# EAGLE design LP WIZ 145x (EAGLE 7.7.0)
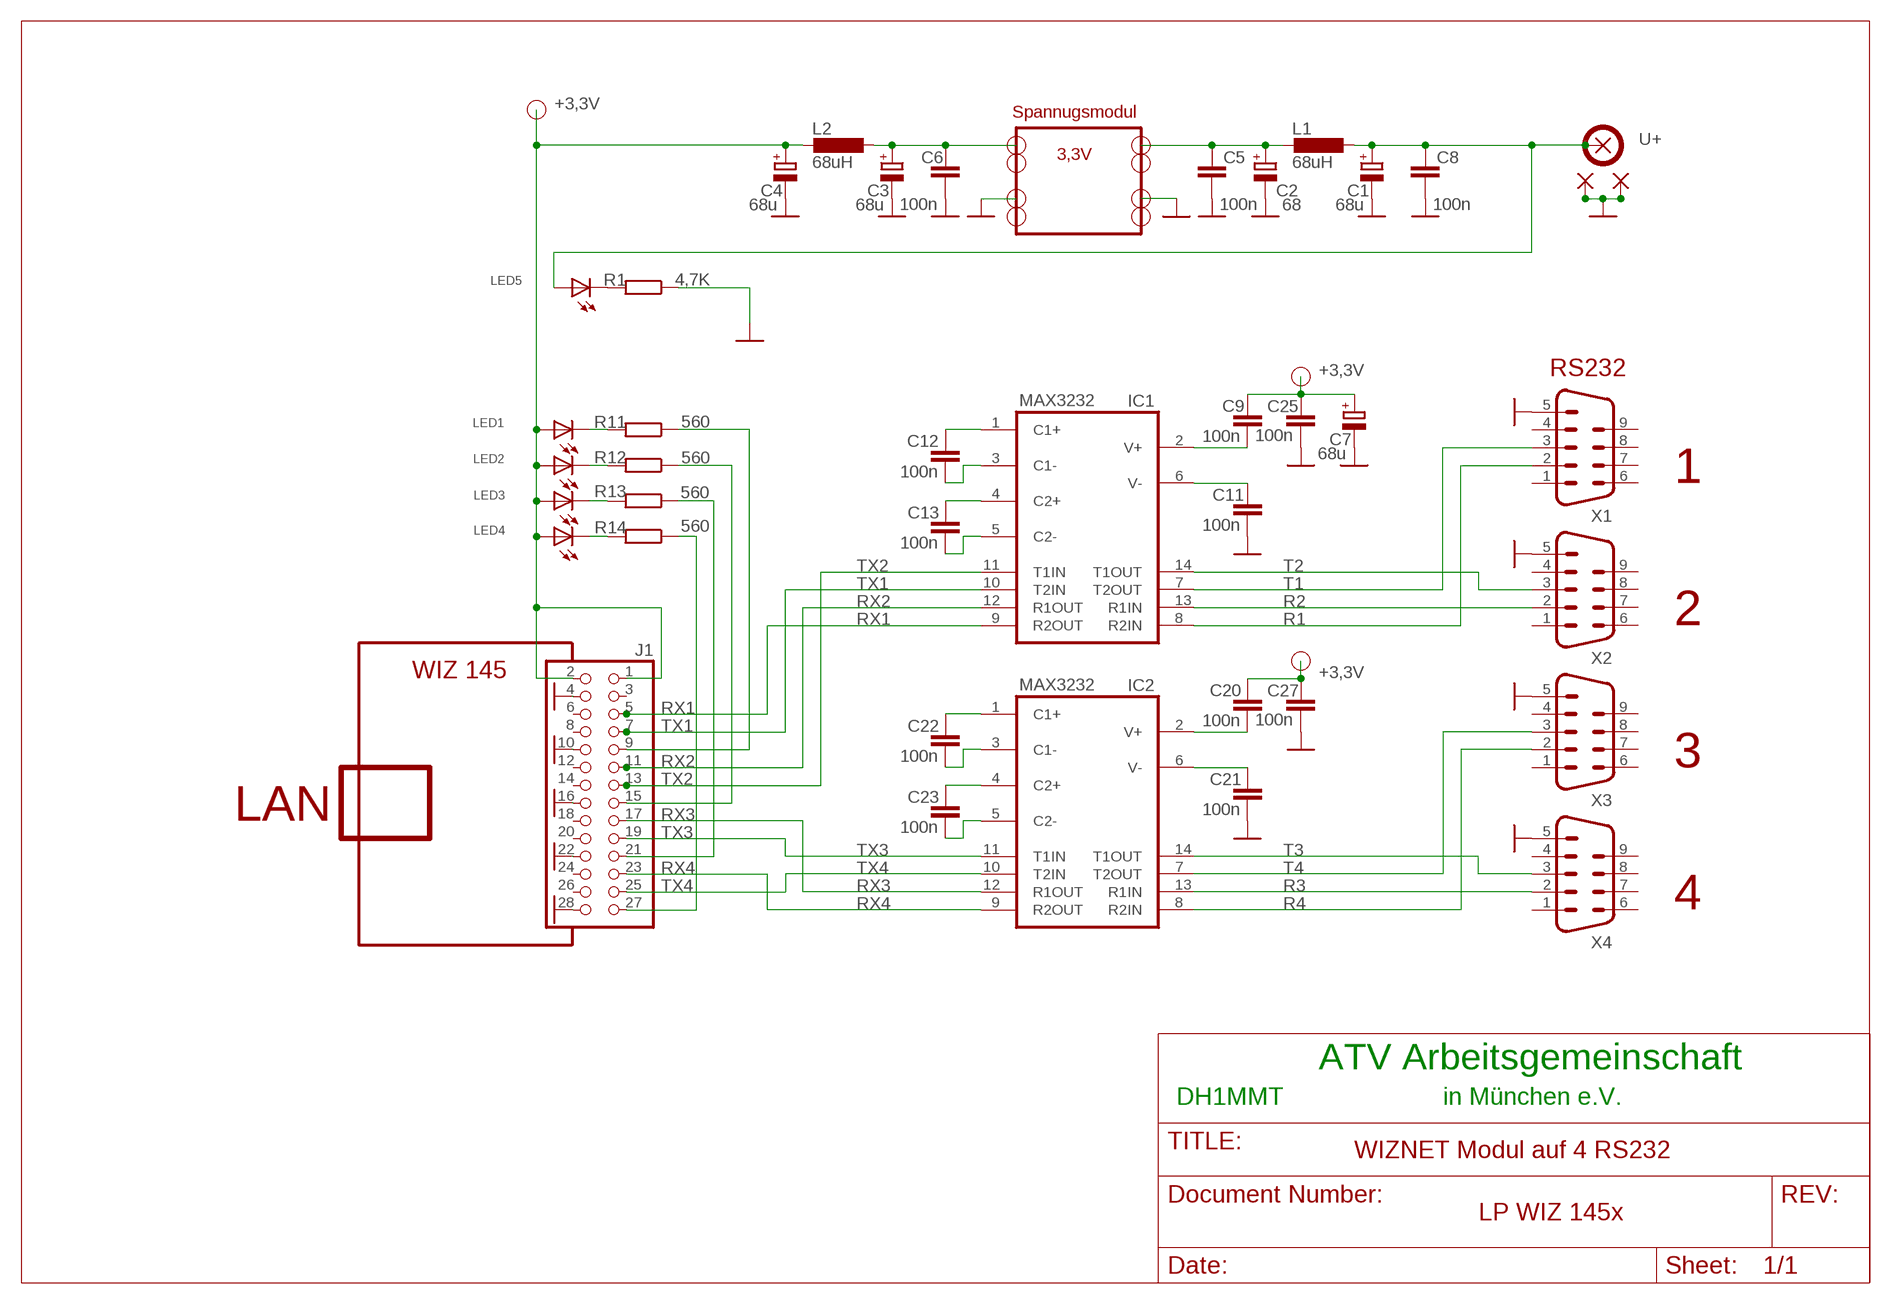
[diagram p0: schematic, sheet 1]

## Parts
C1  68u  CPOL-EUE2.5-5  [E2,5-5]
C2  68  CPOL-EUE2.5-5  [E2,5-5]
C3  68u  CPOL-EUE2.5-5  [E2,5-5]
C4  68u  CPOL-EUE2.5-5  [E2,5-5]
C5  100n  C-EUC0805K  [C0805K]
C6  100n  C-EUC0805K  [C0805K]
C7  68u  CPOL-EUE2.5-5  [E2,5-5]
C8  100n  C-EUC0805K  [C0805K]
C9  100n  C-EUC0805K  [C0805K]
C11  100n  C-EUC0805K  [C0805K]
C12  100n  C-EUC0805K  [C0805K]
C13  100n  C-EUC0805K  [C0805K]
C20  100n  C-EUC0805K  [C0805K]
C21  100n  C-EUC0805K  [C0805K]
C22  100n  C-EUC0805K  [C0805K]
C23  100n  C-EUC0805K  [C0805K]
C25  100n  C-EUC0805K  [C0805K]
C27  100n  C-EUC0805K  [C0805K]
IC1  MAX3232  MAX232  [DIL16]
IC2  MAX3232  MAX232  [DIL16]
J1  PINHD-2X14  [2X14]
L1  68uH  L-EU0207/15  [0207/15]
L2  68uH  L-EU0207/15  [0207/15]
LED1  LED3MM  [LED3MM]
LED2  LED3MM  [LED3MM]
LED3  LED3MM  [LED3MM]
LED4  LED3MM  [LED3MM]
LED5  LED3MM  [LED3MM]
PAD1  SMD5  [SMD2,54-5,08]
PAD2  SMD5  [SMD2,54-5,08]
PAD3  SMD5  [SMD2,54-5,08]
PAD4  SMD5  [SMD2,54-5,08]
PAD6  SMD5  [SMD2,54-5,08]
PAD7  SMD5  [SMD2,54-5,08]
R1  4,7K  R-EU_MELF0204W  [MINI_MELF-0204W]
R11  560  R-EU_MELF0204W  [MINI_MELF-0204W]
R12  560  R-EU_MELF0204W  [MINI_MELF-0204W]
R13  560  R-EU_MELF0204W  [MINI_MELF-0204W]
R14  560  R-EU_MELF0204W  [MINI_MELF-0204W]
X1  M09VP  [M09VP]
X2  M09VP  [M09VP]
X3  M09VP  [M09VP]
X4  M09VP  [M09VP]

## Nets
+3,3V: C4.+ C7.+ C9.2 C20.2 C25.2 C27.2 J1.1 J1.2 L2.2 LED1.A LED2.A LED3.A LED4.A
GND: C1.- C2.- C3.- C4.- C5.1 C6.1 C7.- C8.1 C11.1 C21.1 C25.1 C27.1 J1.4 J1.10 J1.16 J1.22 J1.28 PAD2.1(P) PAD3.1(P) PAD6.1(P) PAD7.1(P) R1.1 X1.5 X2.5 X3.5 X4.5
N$13: LED5.K(C) R1.2
N$15: C3.+ C6.2 L2.1
N$17: C2.+ C5.2 L1.2
N$19: J1.27 R14.1
N$28: C13.2 IC1.4(C2+)
N$29: C13.1 IC1.5(C2-)
N$30: C12.2 IC1.1(C1+)
N$33: C12.1 IC1.3(C1-)
N$35: LED1.K(C) R11.2
N$38: C9.1 IC1.2(V+)
N$39: C11.2 IC1.6(V-)
N$40: J1.21 R13.1
N$43: J1.15 R12.1
N$44: J1.9 R11.1
N$45: LED2.K(C) R12.2
N$46: LED3.K(C) R13.2
N$47: LED4.K(C) R14.2
N$80: C22.2 IC2.1(C1+)
N$82: C22.1 IC2.3(C1-)
N$87: C23.2 IC2.4(C2+)
N$88: C23.1 IC2.5(C2-)
N$91: C21.2 IC2.6(V-)
N$93: C20.1 IC2.2(V+)
R1: IC1.8(R2IN) X1.2
R2: IC1.13(R1IN) X2.2
R3: IC2.13(R1IN) X4.2
R4: IC2.8(R2IN) X3.2
RX1: IC1.9(R2OUT) J1.5
RX2: IC1.12(R1OUT) J1.11
RX3: IC2.12(R1OUT) J1.17
RX4: IC2.9(R2OUT) J1.23
T1: IC1.7(T2OUT) X1.3
T2: IC1.14(T1OUT) X2.3
T3: IC2.14(T1OUT) X4.3
T4: IC2.7(T2OUT) X3.3
TX1: IC1.10(T2IN) J1.7
TX2: IC1.11(T1IN) J1.13
TX3: IC2.11(T1IN) J1.19
TX4: IC2.10(T2IN) J1.25
U+: C1.+ C8.2 L1.1 LED5.A PAD1.1(P) PAD4.1(P)
Unconnected: J1.3 J1.6 J1.8 J1.12 J1.14 J1.18 J1.20 J1.24 J1.26 X1.1 X1.4 X1.6 X1.7 X1.8 X1.9 X2.1 X2.4 X2.6 X2.7 X2.8 X2.9 X3.1 X3.4 X3.6 X3.7 X3.8 X3.9 X4.1 X4.4 X4.6 X4.7 X4.8 X4.9

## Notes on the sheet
- Spannugsmodul
- 3,3V
- RS232
- 1
- 2
- WIZ 145
- 3
- LAN
- 4
- ATV Arbeitsgemeinschaft
- DH1MMT | in München e.V.
- WIZNET Modul auf 4 RS232

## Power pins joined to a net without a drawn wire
+3,3V: IC1.16(VCC) IC2.16(VCC)
GND: IC1.15(GND) IC2.15(GND)

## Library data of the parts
C1-C4 C7 = rcl:CPOL-EU: POLARIZED CAPACITOR, European symbol
C5 C6 C8 C9 C11-C13 C20-C23 C25 C27 = rcl:C-EU: CAPACITOR, European symbol
IC1 IC2 = maxim:MAX232: RS232 TRANSCEIVER; MF: MAXIM; MPN: MAX232ACPE+; OC_FARNELL: 9723773; OC_NEWARK: 68K4544
J1 = pinhead:PINHD-2X14: PIN HEADER
L1 L2 = rcl:L-EU: INDUCTOR, European symbol
LED1-LED5 = led:LED: LED
PAD1-PAD4 PAD6 PAD7 = wirepad:SMD5: SMD PAD
R1 R11-R14 = rcl:R-EU_: RESISTOR, European symbol
X1-X4 = con-subd:M09: SUB-D; OC_FARNELL: unknown; OC_NEWARK: unknown

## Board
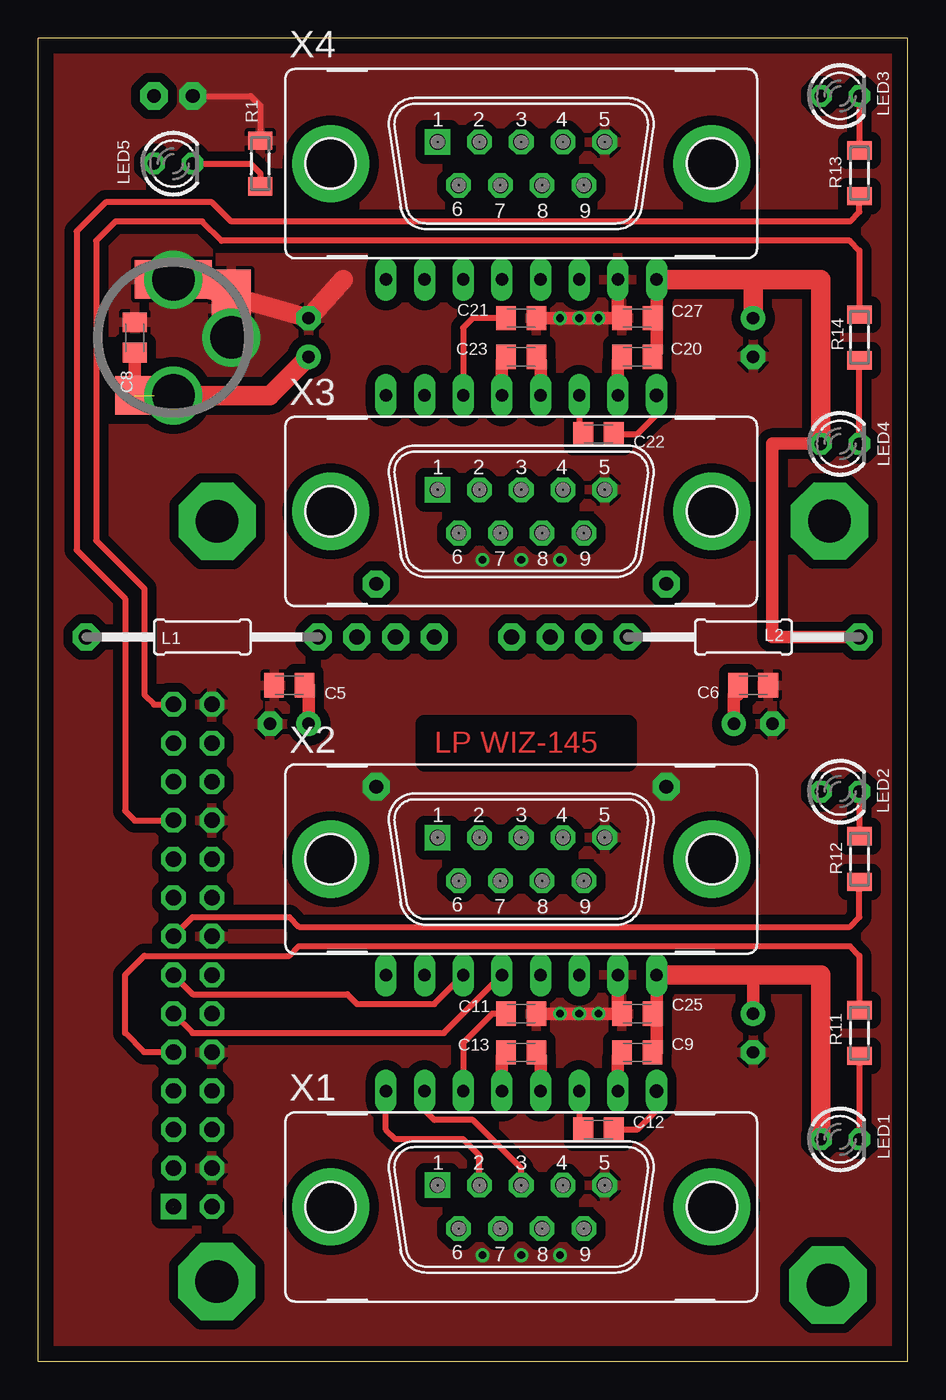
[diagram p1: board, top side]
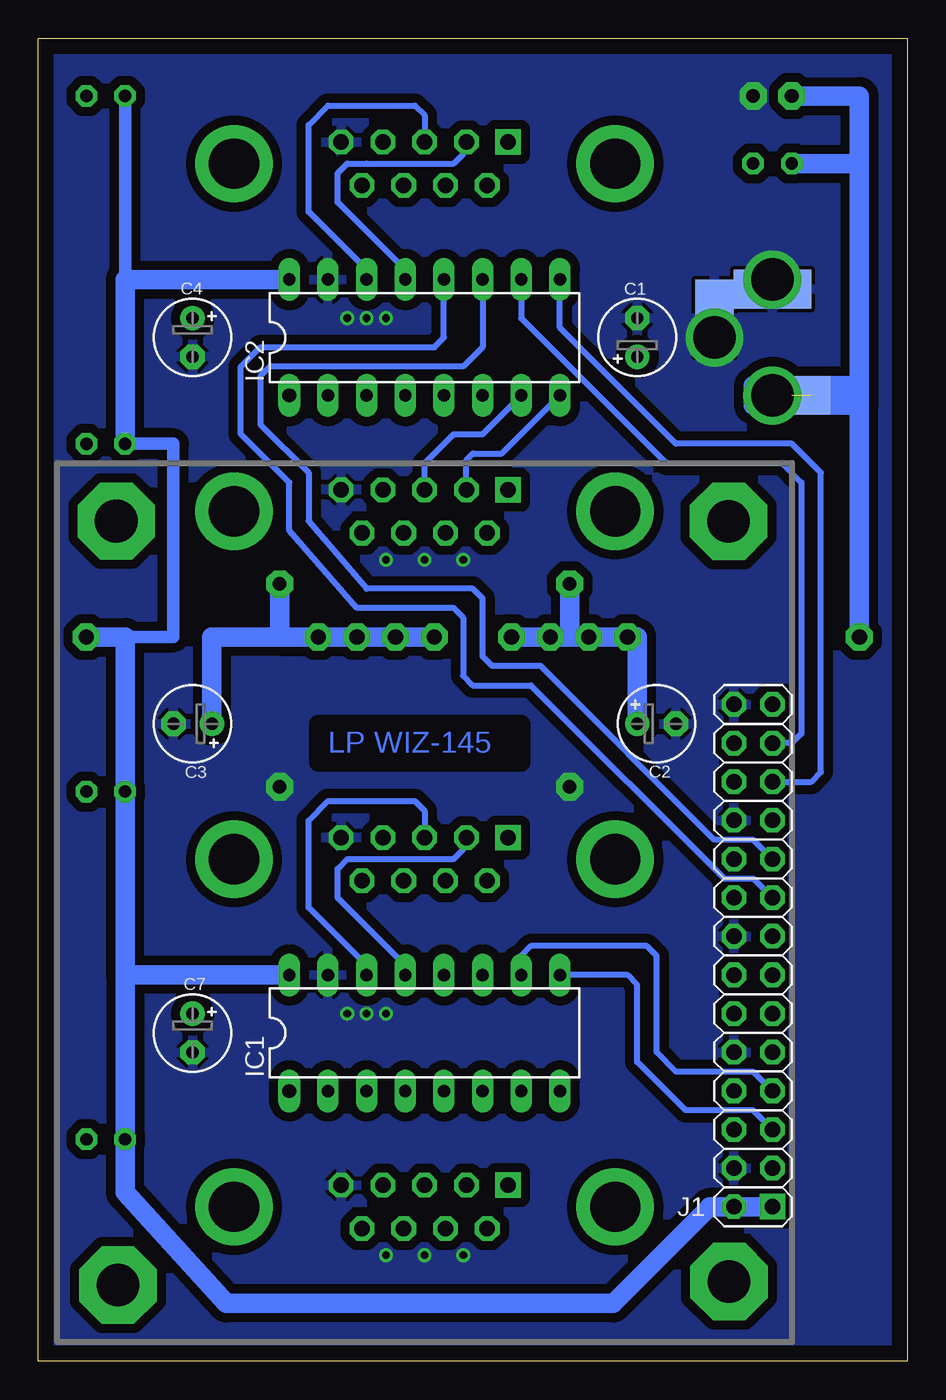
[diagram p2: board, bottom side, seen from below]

Size 57.15 x 87 mm. Coordinates in mm from the lower left corner, seen from the top.
Outline: 57.15,0 57.15,87 0,87 0,0 57.15,0
Copper layers (1*16): Top 0.035mm / dielectric 1.5mm / Bottom 0.035mm
Design rules "default *": minimum track width 10mil, minimum drill 24mil, track to track 20mil, track to pad 20mil, pad to pad 20mil, via to via 20mil, smd to smd 20mil, copper to edge 40mil, drill to drill 8mil, minimum pad ring 0.3mm, minimum via ring 0.2mm, stop-mask expansion 0mil, vias tented up to drill 0mil, thermal gap 10mil
tRestrict: area 25.4,39.4 to 38.7,41.9
bRestrict: area 25.4,39.4 to 38.7,41.9

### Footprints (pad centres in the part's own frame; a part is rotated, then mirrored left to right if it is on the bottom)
E2,5-5 = drill 0.813 pad 1.6: + -1.27,0 | drill 0.813 pad 1.6 octagon: - 1.27,0
C0805K = smd 1.3 x 1.6: 1 -1,0; 2 1,0
DIL16 = drill 0.813 long: 1 -8.89,-3.81; 2 -6.35,-3.81; 3 -3.81,-3.81; 4 -1.27,-3.81; 5 1.27,-3.81; 6 3.81,-3.81; 7 6.35,-3.81; 8 8.89,-3.81; 9 8.89,3.81; 10 6.35,3.81; 11 3.81,3.81; 12 1.27,3.81; 13 -1.27,3.81; 14 -3.81,3.81; 15 -6.35,3.81; 16 -8.89,3.81
2X14 = drill 1.016 octagon: 1 -16.51,-1.27; 2 -16.51,1.27; 3 -13.97,-1.27; 4 -13.97,1.27; 5 -11.43,-1.27; 6 -11.43,1.27; 7 -8.89,-1.27; 8 -8.89,1.27; 9 -6.35,-1.27; 10 -6.35,1.27; 11 -3.81,-1.27; 12 -3.81,1.27; 13 -1.27,-1.27; 14 -1.27,1.27; 15 1.27,-1.27; 16 1.27,1.27; 17 3.81,-1.27; 18 3.81,1.27; 19 6.35,-1.27; 20 6.35,1.27; 21 8.89,-1.27; 22 8.89,1.27; 23 11.43,-1.27; 24 11.43,1.27; 25 13.97,-1.27; 26 13.97,1.27; 27 16.51,-1.27; 28 16.51,1.27
0207/15 = drill 0.813 octagon: 1 -7.62,0; 2 7.62,0
LED3MM = drill 0.813 octagon: A -1.27,0; K 1.27,0
SMD2,54-5,08 = smd 2.54 x 5.08: 1 0,0
MINI_MELF-0204W = smd 1.2 x 1.6: 1 -1.5,0; 2 1.5,0
M09VP = drill 1.016 octagon: 1 -5.486,1.422; 2 -2.743,1.422; 3 0,1.422; 4 2.743,1.422; 5 5.486,1.422; 6 -4.115,-1.422; 7 -1.372,-1.422; 8 1.372,-1.422; 9 4.115,-1.422 | drill 3.302 pad 5.08: G1 -12.522,0; G2 12.522,0

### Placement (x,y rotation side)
C1  17.78,67.31 90 bottom
C2  16.51,41.91 0 bottom
C3  46.99,41.91 180 bottom
C4  46.99,67.31 270 bottom
C5  16.51,44.45 0 top
C6  46.99,44.45 180 top
C7  46.99,21.59 270 bottom
C8  6.35,67.31 270 top
C9  39.37,20.32 0 top
C11  31.75,22.86 180 top
C12  36.83,15.24 0 top
C13  31.75,20.32 0 top
C20  39.37,66.04 0 top
C21  31.75,68.58 180 top
C22  36.83,60.96 0 top
C23  31.75,66.04 0 top
C25  39.37,22.86 0 top
C27  39.37,68.58 0 top
IC1  31.75,21.59 0 bottom
IC2  31.75,67.31 0 bottom
J1  10.16,26.68 90 bottom
L1  10.79,47.62 0 top
L2  46.35,47.62 0 top
LED1  52.7,14.61 0 top
LED2  52.7,37.47 0 top
LED3  52.7,83.19 0 top
LED4  52.7,60.33 0 top
LED5  8.89,78.74 0 top
PAD1  7.62,63.5 270 top
PAD2  12.7,69.22 180 top
PAD3  8.89,71.12 90 top
PAD4  7.62,63.5 90 bottom
PAD6  8.89,70.48 270 bottom
PAD7  12.7,68.58 0 bottom
R1  14.6,78.74 270 top
R11  53.97,21.59 270 top
R12  53.97,33.02 90 top
R13  53.97,78.11 90 top
R14  53.97,67.31 270 top
U$2  [DINA4_L]  not placed on the board
U$3  [DOCFIELD]  not placed on the board
X1  31.75,10.16 0 top
X2  31.75,33.02 0 top
X3  31.75,55.88 0 top
X4  31.75,78.74 0 top

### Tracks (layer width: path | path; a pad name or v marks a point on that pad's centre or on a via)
+3,3V  (1 unrouted)
  Top 0.813: IC1.16 40.64,23.13 C25.2 | C9.2 40.64,20.32 IC1.16 | 40.64,22.86 IC1.16 | 46.99,25.4 C7.+ | 40.64,68.58 IC2.16 40.64,68.85 C27.2 40.64,68.58 | 40.64,68.58 40.64,66.31 C20.2 | LED4.A 48.26,60.33 48.26,47.62 L2.2
  Top 1.27: IC1.16 46.99,25.4 51.44,25.4 LED1.A | IC2.16 46.99,71.12 | C4.+ 46.99,71.12 | 46.99,71.12 51.44,71.12 LED4.A
  Bottom 0.813: 51.44,47.62 48.26,47.62 48.26,60.33 LED4.A | 51.44,71.12 LED3.A | J1.1 J1.2
  Bottom 1.27: LED4.A 51.44,71.12 IC2.16 | L2.2 51.44,47.62 LED2.A 51.44,25.4 | IC1.16 51.44,25.4 | 51.44,25.4 LED1.A 51.44,11.11 44.77,3.81 19.37,3.81 13.02,10.16 J1.1
GND  (via drill 0.5, 0.9 pad 1.78, 2.8 pad 3.81)
  Top 0.406: v10.16,83.19 13.97,83.19 14.6,82.55 R1.1
  Top 0.813: IC1.15 38.1,23.13 C25.1 C11.1 | IC2.15 38.1,68.85 C27.1 v36.83,68.58 v35.56,68.58 v34.29,68.58 C21.1
  Top 1.27: 20.05,71.12 C1.- PAD3.1 9.52,70.48 13.33,70.48
  other vias: 41.27,37.78 22.22,37.78 36.83,22.86 34.29,22.86 35.56,22.86 8.89,71.12 12.7,67.31 31.75,6.98 34.29,6.98 29.21,6.98 31.75,52.7 34.29,52.7 29.21,52.7
  pour Top (isolate 0.61): -5.08,-2.54 60.96,-2.54 60.96,88.9 -5.08,88.9
  pour Bottom (isolate 0.61): -5.08,-2.54 60.96,-2.54 60.96,88.9 -5.08,88.9
N$1  (via drill 1 pad 1.78)
  other vias: 18.41,47.62
N$3  (via drill 1 pad 1.78)
  other vias: 38.73,47.62
N$6  (via drill 1 pad 1.78)
  other vias: 53.97,47.62
N$11  (via drill 1 pad 1.78)
  other vias: 3.17,47.62
N$12
  Bottom 0.406: 35.56,78.74 29.84,78.74
N$13
  Top 0.406: LED5.K 13.97,78.74 14.6,78.11 R1.2
N$15  (via drill 0.8 pad 1.42, 0.9 pad 1.78, 1 pad 1.78)
  Top 0.813: C3.+ 45.72,43.81 45.99,43.81 C6.2
  Bottom 1.27: L2.1 41.27,47.62 41.27,48.58 41.27,48.89 41.27,49.53 v41.27,51.12 | L2.1 v36.19,47.62 v33.66,47.62 v31.11,47.62 | L2.1 45.72,47.62 C3.+
  other vias: 38.73,47.62
N$17  (via drill 0.9 pad 1.78, 1 pad 1.78)
  Top 0.813: C2.+ 17.78,44.45 C5.2
  Bottom 1.27: 22.22,47.62 v23.49,47.62 v26.03,47.62 | 22.22,47.62 21.59,47.62 v20.95,47.62 L1.2 17.78,47.62 C2.+ | v22.22,51.12 22.22,47.62
N$18  (via drill 0.8 pad 1.42)
  other vias: 18.41,47.62
N$19
  Top 0.406: J1.27 7.62,43.18 6.98,43.81 6.98,50.8 3.81,53.97 3.81,73.66 5.08,74.93 10.79,74.93 12.06,73.66 53.34,73.66 53.97,73.03 R14.1
N$21  (via drill 0.9 pad 1.42)
  other vias: 40.64,17.78
N$22  (via drill 0.9 pad 1.42)
  other vias: 40.64,63.5
N$24  (via drill 1 pad 1.68)
  other vias: 26.26,57.3
N$25  (via drill 1 pad 1.68)
  other vias: 26.26,80.17
N$26  (via drill 1 pad 1.68)
  other vias: 26.26,34.44
N$28
  Top 0.813: IC1.4 33.02,20.05 C13.2
N$29
  Top 0.813: IC1.5 30.48,20.05 C13.1
N$30
  Top 0.406: IC1.1 40.64,16.51 39.37,15.24 C12.2
N$31  (via drill 1 pad 1.68)
  other vias: 26.26,11.59
N$32  (via drill 1 pad 1.68)
  other vias: 8.9,10.18
N$33
  Top 0.406: IC1.3 35.56,15.88 36.19,15.24 C12.1
N$35
  Top 0.406: R11.2 LED1.K
N$38
  Top 0.813: IC1.2 38.1,20.05 C9.1
N$39
  Top 0.406: C11.2 29.84,22.86 27.94,20.95 IC1.6
N$40
  Top 0.406: J1.21 6.35,35.56 5.72,36.2 5.72,50.17 2.54,53.34 2.54,74.3 4.44,76.2 11.43,76.2 12.7,74.93 53.34,74.93 53.97,75.56 R13.1
N$43
  Top 0.406: J1.15 10.16,29.21 16.51,29.21 17.14,28.58 53.34,28.58 53.97,29.21 R12.1
N$44
  Top 0.406: J1.9 6.98,20.33 5.72,21.59 5.72,25.4 6.98,26.67 16.51,26.67 17.14,27.31 53.34,27.31 53.97,26.67 R11.1
N$45
  Top 0.406: LED2.K R12.2
N$46
  Top 0.406: LED3.K R13.2
N$47
  Top 0.406: LED4.K R14.2
N$80
  Top 0.406: C22.2 39.37,60.96 40.64,62.23 IC2.1
N$82
  Top 0.406: IC2.3 35.56,61.23 C22.1
N$87
  Top 0.813: IC2.4 33.02,65.77 C23.2
N$88
  Top 0.813: IC2.5 30.48,65.77 C23.1
N$91
  Top 0.406: C21.2 28.57,68.58 27.94,67.95 IC2.6
N$93
  Top 0.813: IC2.2 38.1,65.77 C20.1
N$94  (via drill 2.8 pad 5.08)
  other vias: 11.77,55.23
N$96  (via drill 2.8 pad 5.08)
  other vias: 52.01,55.24
N$97  (via drill 2.8 pad 5.08)
  other vias: 11.74,5.25
N$98  (via drill 2.8 pad 5.08)
  other vias: 51.9,5.02
R1
  Top 0.406: IC1.8 22.86,15.24 23.49,14.61 27.94,14.61 29.01,13.54 X1.2
R2
  Bottom 0.406: IC1.13 33.02,26.03 37.47,30.48 37.47,32.39 36.83,33.02 29.84,33.02 29.21,33.66 29.21,34.24 X2.2
R3
  Bottom 0.406: IC2.13 33.02,71.75 37.47,76.2 37.47,78.11 36.83,78.74 29.84,78.74 29.21,79.38 29.21,79.96 X4.2
R4
  Bottom 0.406: IC2.8 26.67,59.69 28.57,59.69 29.01,59.26 X3.2
RX1
  Bottom 0.406: J1.5 10.16,16.51 14.6,16.51 17.78,19.69 17.78,24.77 18.41,25.4 IC1.9
RX2
  Top 0.406: J1.11 10.16,21.59 26.67,21.59 IC1.12
RX3
  Bottom 0.406: J1.17 10.15,31.75 12.06,31.75 24.76,44.45 28.57,44.45 29.21,45.09 29.21,48.89 29.84,49.53 36.19,49.53 40.64,54.61 40.64,57.78 43.81,60.96 43.81,65.41 42.54,66.67 31.11,66.67 30.48,67.31 IC2.12
RX4
  Bottom 0.406: J1.23 6.34,38.11 5.72,38.73 5.72,58.42 7.62,60.33 15.24,60.33 22.86,67.95 IC2.9
T1
  Top 0.406: IC1.7 25.4,16.51 26.03,15.88 28.57,15.88 31.75,12.7 X1.3
T2
  Bottom 0.406: IC1.14 35.56,26.03 39.37,29.84 39.37,35.56 38.1,36.83 32.38,36.83 31.75,36.2 X2.3
T3
  Bottom 0.406: IC2.14 35.56,71.75 39.37,75.56 39.37,81.28 38.1,82.55 32.38,82.55 31.75,81.92 X4.3
T4
  Bottom 0.406: IC2.7 27.94,60.96 29.84,60.96 31.75,59.06 X3.3
TX1
  Bottom 0.406: J1.7 10.16,19.05 15.24,19.05 16.51,20.32 16.51,26.67 17.14,27.31 24.76,27.31 25.4,26.67 IC1.10
TX2
  Top 0.406: J1.13 10.16,24.13 20.32,24.13 20.95,23.5 26.03,23.5 IC1.11
TX3
  Bottom 0.406: J1.19 10.16,34.29 12.7,34.29 24.13,45.72 27.3,45.72 27.94,46.36 27.94,50.17 28.57,50.8 35.56,50.8 39.37,55.25 39.37,58.42 42.54,61.59 42.54,64.77 41.91,65.41 29.21,65.41 27.94,66.67 IC2.11
TX4
  Bottom 0.406: IC2.10 25.4,68.58 15.88,59.06 8.25,59.06 6.98,57.78 6.98,41.28 7.62,40.64 J1.25
U+  (via drill 0.9 pad 1.78, 2.8 pad 3.81)  (2 unrouted)
  Top 0.813: C8.2 6.35,63.5 v8.89,63.5
  Top 1.27: v8.89,63.5 15.24,63.5 C1.+
  Bottom 1.27: L1.1 3.17,62.86 | 3.17,62.86 4.44,63.5 | 4.44,63.5 v8.89,63.5 10.16,63.5 | 3.17,62.86 10.16,62.86 10.16,64.14 3.17,64.14 | 3.17,64.14 4.44,63.5 | v7.62,83.19 3.17,83.19 3.17,78.74 | 3.17,78.74 3.17,64.14 | 3.17,64.14 3.17,62.86 | LED5.A 3.17,78.74

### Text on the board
Top: LP WIZ-145
Bottom: LP WIZ-145
Document: ATV - Arbeitsgemeinschaft | DH1MMT | in München e.V.
tDocu: U+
